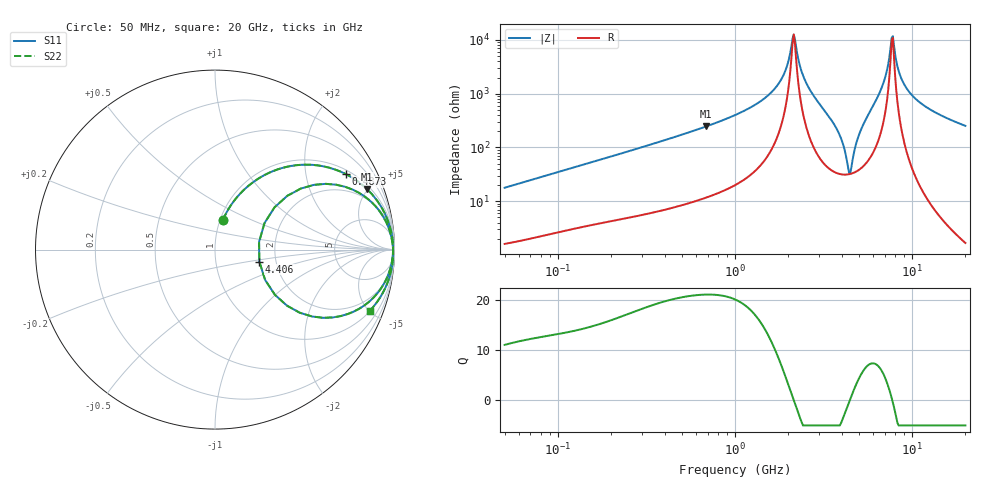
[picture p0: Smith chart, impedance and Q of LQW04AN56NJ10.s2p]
!Murata Part Number: LQW04AN56NJ10
!These Parameters are Measured in Series Mode Connection
!  o--[Z]--o
!Port1  Port2
!  o-------o
!Freq. Start=50[MHz] Stop=20[GHz], 401[Steps]
# Hz S RI R 50
!Freq.(Hz) S11(Real) S11(Imag) S21(Real) S21(Imag) S12(Real) S12(Imag) S22(Real) S22(Imag)
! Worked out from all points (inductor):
!   401 points, 50 MHz to 20 GHz, reference 50 ohm
!   read as one part in series: L = 56 nH near 51.52 MHz
!   highest Q = 21.1 at 687.7 MHz (marker M1), where L = 56.9 nH
!   self-resonance near 2.115 GHz
!   S11 on the Smith chart (normalised r, x): 50 MHz: 1.03, +0.35; 487.3 MHz: 1.16, +3.35; 4.406 GHz: 1.64, -0.23; 20 GHz: 1.03, -5.04
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5e7  0.0449 0.1666  0.9551 -0.1666  0.9551 -0.1666  0.0449 0.1666
1.364002e8  0.1969 0.364  0.8031 -0.364  0.8031 -0.364  0.1969 0.364
3.721004e8  0.6101 0.4626  0.3899 -0.4626  0.3899 -0.4626  0.6101 0.4626
4.872511e8  0.7281 0.4212  0.2719 -0.4212  0.2719 -0.4212  0.7281 0.4212
6.87656e8  0.847 0.3371  0.153 -0.3371  0.153 -0.3371  0.847 0.3371
1e9  0.931 0.2299  0.069 -0.2299  0.069 -0.2299  0.931 0.2299
1.714689e9  0.9871 0.0717  0.0129 -0.0717  0.0129 -0.0717  0.9871 0.0717
1.932977e9  0.9912 0.0346  0.0088 -0.0346  0.0088 -0.0346  0.9912 0.0346
2.146657e9  0.9921 -2.13e-05  0.00785 2.13e-05  0.00785 2.13e-05  0.9921 -2.13e-05
2.419936e9  0.9892 -0.0438  0.0108 0.0438  0.0108 0.0438  0.9892 -0.0438
2.728004e9  0.9795 -0.0955  0.0205 0.0955  0.0205 0.0955  0.9795 -0.0955
3.466789e9  0.8957 -0.2539  0.1043 0.2539  0.1043 0.2539  0.8957 -0.2539
3.967106e9  0.6562 -0.378  0.3438 0.378  0.3438 0.378  0.6562 -0.378
4.405649e9  0.247 -0.0668  0.753 0.0668  0.753 0.0668  0.247 -0.0668
4.89267e9  0.6176 0.3663  0.3824 -0.3663  0.3824 -0.3663  0.6176 0.3663
5.433528e9  0.8751 0.2616  0.1249 -0.2616  0.1249 -0.2616  0.8751 0.2616
6.601595e9  0.9784 0.0865  0.0216 -0.0865  0.0216 -0.0865  0.9784 0.0865
7.442007e9  0.9907 0.0185  0.0093 -0.0185  0.0093 -0.0185  0.9907 0.0185
7.784049e9  0.9921 -0.0031  0.00785 0.0031  0.00785 0.0031  0.9921 -0.0031
8.774992e9  0.9911 -0.0547  0.0089 0.0547  0.0089 0.0547  0.9911 -0.0547
1.050288e10  0.9803 -0.1228  0.0197 0.1228  0.0197 0.1228  0.9803 -0.1228
2e10  0.8624 -0.3412  0.1376 0.3412  0.1376 0.3412  0.8624 -0.3412
